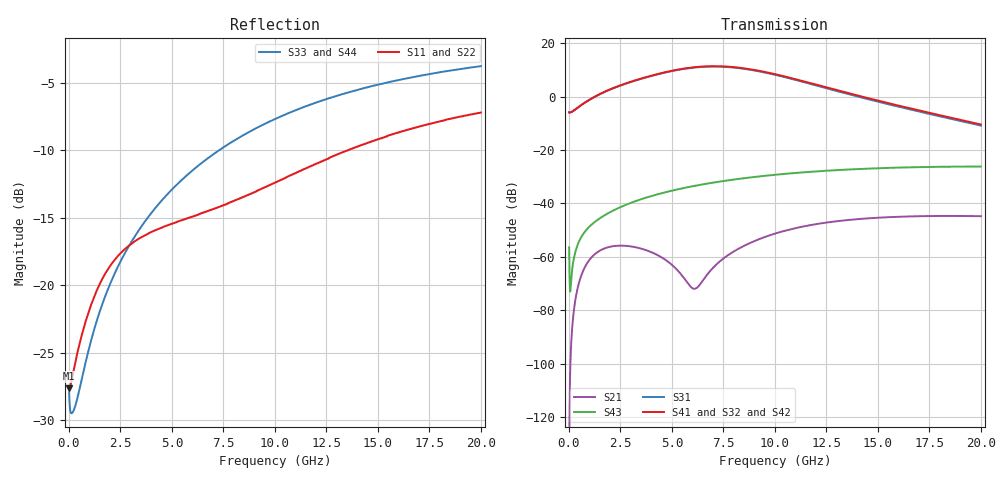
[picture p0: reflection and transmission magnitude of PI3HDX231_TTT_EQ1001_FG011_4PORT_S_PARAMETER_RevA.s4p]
! NPort=4 DATA=2000 NOISE=0 GROUPDELAY=0 COMPLEX_DATAFORMAT=POLAR
! NumOfBlock=1 NumOfParam=0
! .MODEL Smodel S TSTONEFILE=PI3HDX231_TTT_EQ1001_FG011_4PORT_S_PARAMETER_RevA.s4p TYPE=S
!  -- The above .MODEL line can be used for the S element in the netlist.
! The s parameter is extracted from the linear redriver, it is not bi-directional; only s(4,1)s(4,2) and s(3,1)s(3,2)
! should be the insertion loss
!Port definition:
!Port1 = input+
!Port2 = input-
!Port3 = output+
!Port4 = output-
# Hz S MA R  50
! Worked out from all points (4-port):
!   2000 points, 10 MHz to 20 GHz, reference 50 ohm
!   strongest paths, dB at 10 MHz, 5.01 GHz, 10.01 GHz, 15.01 GHz, 20 GHz:
!     S41: -5.9, 9.7, 8.4, -1.5, -10.5
!     S32: -5.9, 9.6, 8.3, -1.5, -10.4
!     S42: -5.9, 9.7, 8.3, -1.7, -10.6
!     S31: -5.9, 9.6, 8.1, -1.9, -10.9
!     S43: -56.5, -35.2, -29.3, -26.8, -26.2
!     S21: -134.8, -63.1, -51.3, -45.4, -44.8
!   lowest |S11| = -27.6 dB at 10 MHz (marker M1), VSWR 1.09, Z = 46 - j0.0776 ohm
!   |S11| at or under -10 dB: start of sweep to 13.55 GHz
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1e7  0.04152 -178.8  1.825e-07 -14.0  0 0.0  0 0.0
     1.825e-07 -13.9  0.04152 -178.8  0 0.0  0 0.0
     0.5042 -0.1  0.5042 179.9  0.04012 -3.2  0.0015 -70.3
     0.5042 179.9  0.5042 -0.1  0.0015 -70.3  0.04012 -3.2
4.39e9  0.1621 -140.7  0.001031 -8.7  2.855e-10 -154.1  1.883e-10 -137.7
        0.001031 -8.6  0.1621 -140.9  1.778e-10 -138.0  3.003e-10 -153.4
        2.657 -45.5  2.662 134.2  0.2011 -100.6  0.01512 64.8
        2.688 134.3  2.685 -44.7  0.01509 64.7  0.2011 -100.6
6.33e9  0.1835 -137.5  0.0002858 69.8  2.648e-09 143.9  1.488e-09 -177.9
        0.0002925 69.2  0.1832 -137.7  1.403e-09 -176.3  2.801e-09 143.5
        3.56 -105.3  3.576 74.4  0.2791 -106.3  0.02215 53.9
        3.612 74.3  3.608 -104.4  0.02208 53.9  0.2792 -106.3
8.22e9  0.2085 -132.9  0.001405 98.9  1.148e-08 85.1  7.817e-09 134.6
        0.001405 98.4  0.2078 -133.2  7.504e-09 137.2  1.211e-08 83.7
        3.414 -169.0  3.453 10.7  0.3502 -111.3  0.02875 42.1
        3.484 10.4  3.468 -168.1  0.02865 42.2  0.3503 -111.3
1.067e10  0.2533 -128.8  0.003211 77.6  4.07e-08 19.2  3.335e-08 62.0
          0.003204 77.3  0.2519 -129.0  3.262e-08 64.8  4.231e-08 16.8
          2.211 118.7  2.265 -61.8  0.4338 -117.3  0.03628 26.1
          2.279 -62.3  2.251 119.9  0.03618 26.3  0.4338 -117.3
1.364e10  0.3178 -128.4  0.004933 46.9  1.132e-07 -47.4  9.294e-08 -15.8
          0.004914 46.6  0.3158 -128.4  9.251e-08 -13.1  1.154e-07 -50.0
          1.091 54.1  1.138 -127.4  0.5192 -123.8  0.04321 6.7
          1.139 -128.1  1.117 55.4  0.04316 7.0  0.5191 -123.8
2e10  0.4355 -135.6  0.00578 -4.2  3.763e-07 -160.7  2.811e-07 -140.4
      0.00575 -4.4  0.4338 -135.4  2.845e-07 -138.9  3.75e-07 -162.9
      0.2861 -45.5  0.3022 129.1  0.6464 -135.0  0.04883 -32.3
      0.2997 128.8  0.2965 -44.1  0.04895 -32.1  0.6461 -135.0
